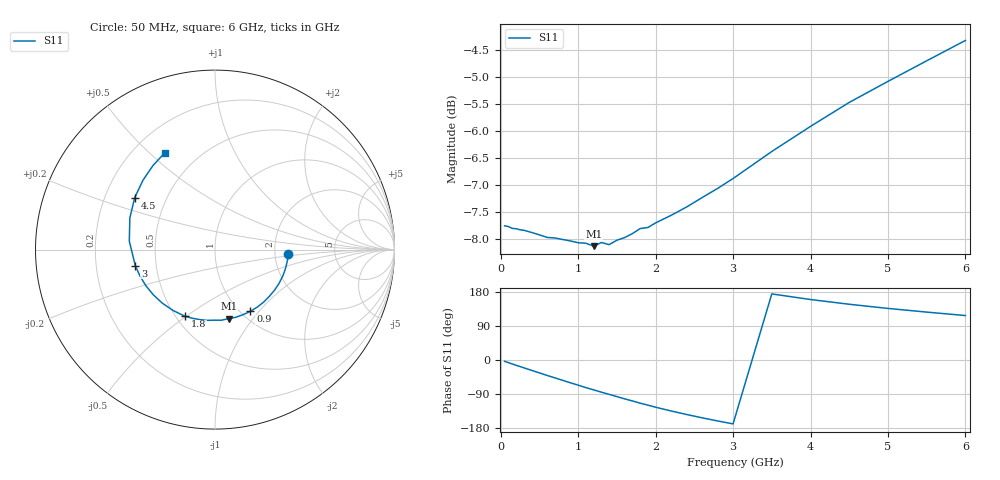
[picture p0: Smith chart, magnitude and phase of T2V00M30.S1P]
! SIEMENS Discrete & RF Semiconductors
! BAS70-04W
! Si Schottky Diode in SOT323
! IF = 0.3 mA
! S-Parameters:  November  1997
# GHz  S  MA  R  50
!  f  S11
! GHz  MAG  ANG
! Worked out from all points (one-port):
!   34 points, 50 MHz to 6 GHz, reference 50 ohm
!   lowest |S11| = -8.1 dB at 1.2 GHz (marker M1), VSWR 2.29, Z = 42.3 - j38.4 ohm
!   |S11| at or under -10 dB: nowhere
!   S11 on the Smith chart (normalised r, x): 50 MHz: 2.38, -0.15; 900 MHz: 1.10, -0.90; 1.8 GHz: 0.56, -0.50; 3 GHz: 0.38, -0.09; 4.5 GHz: 0.33, +0.27; 6 GHz: 0.33, +0.56
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0.05  0.4094 -3.6
0.1  0.4087 -7.0
0.25  0.4059 -17.3
0.4  0.4036 -27.4
0.5  0.4016 -34.1
0.6  0.3993 -40.8
0.7  0.3989 -47.2
0.8  0.3976 -53.7
0.9  0.3964 -60.2
1.1  0.3944 -72.9
1.2  0.392 -78.8
1.3  0.395 -84.9
1.4  0.3933 -90.7
1.5  0.397 -96.6
1.6  0.3992 -102.6
1.8  0.407 -113.9
2  0.4119 -124.6
2.2  0.4186 -134.5
2.4  0.4261 -143.8
2.6  0.4348 -152.6
2.8  0.4434 -160.8
3  0.4528 -168.6
3.5  0.4797 174.4
4  0.5061 159.6
4.5  0.5327 147.1
5  0.5572 136.1
5.5  0.5822 126.4
6  0.608 117.3
